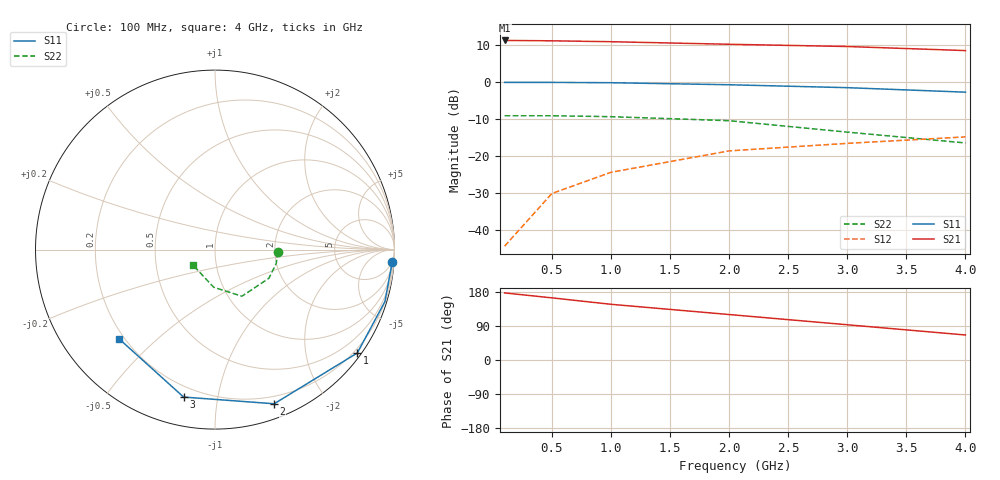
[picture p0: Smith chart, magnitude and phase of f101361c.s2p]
!ATF-10136 / ATF-10135
!S-PARAMETERS at Vds=1V  Id=10mA.  LAST UPDATED 06-28-94
# ghz s ma r 50
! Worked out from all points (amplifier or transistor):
!   6 points, 100 MHz to 4 GHz, reference 50 ohm
!   highest |S21| = 11.3 dB at 100 MHz (marker M1)
!   |S21| within 3 dB of that: start of sweep to end of sweep
!   unconditionally stable (mu >= 1): nowhere
!   at 500 MHz: K = 0.11, MSG = 20.7 dB, |S12| = -30.2 dB
!   at 2 GHz: K = 0.27, MSG = 14.4 dB, |S12| = -18.6 dB
!   at 4 GHz: K = 0.60, MSG = 11.7 dB, |S12| = -14.8 dB
!   lowest NFmin = 0.40 dB at 500 MHz
!   S11 on the Smith chart (normalised r, x): 100 MHz: 4, -28; 1 GHz: 0.11, -3.07; 2 GHz: 0.13, -1.45; 3 GHz: 0.14, -0.80; 4 GHz: 0.18, -0.38
0.1  0.99 -4.0  3.66 177.0  0.006 83.0  0.35 -2.0
0.5  0.99 -17.0  3.62 164.0  0.031 80.0  0.35 -13.0
1  0.98 -36.0  3.52 147.0  0.06 66.0  0.34 -28.0
2  0.92 -69.0  3.25 120.0  0.117 44.0  0.3 -60.0
3  0.84 -102.0  3.03 93.0  0.148 28.0  0.21 -92.0
4  0.73 -137.0  2.67 66.0  0.181 9.0  0.15 -145.0
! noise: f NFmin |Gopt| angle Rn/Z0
0.5  0.4  0.93  12  0.85
1  0.4  0.85  24  0.7
2  0.4  0.7  47  0.46
4  0.5  0.39  126  0.36
